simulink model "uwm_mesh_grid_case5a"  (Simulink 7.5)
settings: Solver=ode45  StartTime=0.0  StopTime=3.0  RelTol=1e-4
undefined symbols (not defined in the file or in its folder): D1, Delta, dfilt, DiscIntNeverNeededParam, Discrete, no, powergui, steady, ZData
libraries: powerlib x259, powerlib_extras x68, dsparch4 x11
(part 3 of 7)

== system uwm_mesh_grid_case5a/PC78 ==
  3-phase  Instantaneous  Active & Reactive Power : powerlib_extras/Measurements/3-phase  Instantaneous  Active & Reactive Power  DialogController=POWERSYS.PowerSysDialog  SystemSampleTime=-1
  Ground : powerlib/Elements/Ground  DialogController=POWERSYS.PowerSysDialog  PhysicalDomain=powersysdomain  SubClassName=unknown  LeftPortType=p1  RightPortType=p1  LConnTagsString=a
  Three-Phase Parallel RLC Branch : powerlib/Elements/Three-Phase Parallel RLC Branch  DialogController=POWERSYS.PowerSysDialog  PhysicalDomain=powersysdomain  SubClassName=unknown  LeftPortType=p1  RightPortType=p1  LConnTagsString=A|B|C  RConnTagsString=A|B|C  BranchType=C  Resistance=1  Inductance=1e-3  Capacitance=1/(C*2*pi*60)  Measurements=None
  Three-Phase Series RLC Branch3 : powerlib/Elements/Three-Phase Series RLC Branch  DialogController=POWERSYS.PowerSysDialog  PhysicalDomain=powersysdomain  SubClassName=unknown  LeftPortType=p1  RightPortType=p1  LConnTagsString=A|B|C  RConnTagsString=A|B|C  BranchType=RL  Resistance=R  Inductance=L/(2*pi*60)  Capacitance=1/(336*2*pi*60)  Measurements=None
  Three-Phase V-I Measurement : powerlib/Measurements/Three-Phase V-I Measurement  DialogController=POWERSYS.PowerSysDialog  SystemSampleTime=-1  VoltageMeasurement=phase-to-ground  SetLabelV=off  LabelV=Vabc  Vpu=off  VpuLL=off  CurrentMeasurement=yes  SetLabelI=off  LabelI=Iabc  Ipu=off  Pbase=100e6  Vbase=500e3  OutputType=Complex  PhasorSimulation=off  PSBequivalent=0
  A* : PMIOPort  Tag=PMCPort  Port=1  Side=Right
  B* : PMIOPort  Tag=PMCPort  Port=2  Side=Right
  C* : PMIOPort  Tag=PMCPort  Port=3  Side=Right
  A : PMIOPort  Tag=PMCPort  Port=4  Side=Left
  B : PMIOPort  Tag=PMCPort  Port=5  Side=Left
  C : PMIOPort  Tag=PMCPort  Port=6  Side=Left
  PQ : Outport  OutDataType=fixdt(1, 16)  OutScaling=2^0
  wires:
  Three-Phase V-I Measurement/1 -> 3-phase  Instantaneous  Active & Reactive Power/1
  Three-Phase V-I Measurement/2 -> 3-phase  Instantaneous  Active & Reactive Power/2
  3-phase  Instantaneous  Active & Reactive Power/1 -> PQ/1
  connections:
  Three-Phase Parallel RLC Branch/LConn1 -- A*/RConn1 -- Three-Phase Series RLC Branch3/LConn1
  Three-Phase Parallel RLC Branch/LConn2 -- B*/RConn1 -- Three-Phase Series RLC Branch3/LConn2
  Three-Phase Parallel RLC Branch/LConn3 -- C*/RConn1 -- Three-Phase Series RLC Branch3/LConn3
  Ground/LConn1 -- Three-Phase Parallel RLC Branch/RConn2 -- Three-Phase Parallel RLC Branch/RConn1 -- Three-Phase Parallel RLC Branch/RConn3
  Three-Phase V-I Measurement/RConn2 -- Three-Phase Series RLC Branch3/RConn2
  Three-Phase V-I Measurement/RConn3 -- Three-Phase Series RLC Branch3/RConn3
  Three-Phase V-I Measurement/RConn1 -- Three-Phase Series RLC Branch3/RConn1
  A/RConn1 -- Three-Phase V-I Measurement/LConn1
  B/RConn1 -- Three-Phase V-I Measurement/LConn2
  C/RConn1 -- Three-Phase V-I Measurement/LConn3

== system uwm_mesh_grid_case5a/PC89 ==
  3-phase  Instantaneous  Active & Reactive Power : powerlib_extras/Measurements/3-phase  Instantaneous  Active & Reactive Power  DialogController=POWERSYS.PowerSysDialog  SystemSampleTime=-1
  Ground : powerlib/Elements/Ground  DialogController=POWERSYS.PowerSysDialog  PhysicalDomain=powersysdomain  SubClassName=unknown  LeftPortType=p1  RightPortType=p1  LConnTagsString=a
  Three-Phase Parallel RLC Branch : powerlib/Elements/Three-Phase Parallel RLC Branch  DialogController=POWERSYS.PowerSysDialog  PhysicalDomain=powersysdomain  SubClassName=unknown  LeftPortType=p1  RightPortType=p1  LConnTagsString=A|B|C  RConnTagsString=A|B|C  BranchType=C  Resistance=1  Inductance=1e-3  Capacitance=1/(C*2*pi*60)  Measurements=None
  Three-Phase Series RLC Branch3 : powerlib/Elements/Three-Phase Series RLC Branch  DialogController=POWERSYS.PowerSysDialog  PhysicalDomain=powersysdomain  SubClassName=unknown  LeftPortType=p1  RightPortType=p1  LConnTagsString=A|B|C  RConnTagsString=A|B|C  BranchType=RL  Resistance=R  Inductance=L/(2*pi*60)  Capacitance=1/(336*2*pi*60)  Measurements=None
  Three-Phase V-I Measurement : powerlib/Measurements/Three-Phase V-I Measurement  DialogController=POWERSYS.PowerSysDialog  SystemSampleTime=-1  VoltageMeasurement=phase-to-ground  SetLabelV=off  LabelV=Vabc  Vpu=off  VpuLL=off  CurrentMeasurement=yes  SetLabelI=off  LabelI=Iabc  Ipu=off  Pbase=100e6  Vbase=500e3  OutputType=Complex  PhasorSimulation=off  PSBequivalent=0
  A* : PMIOPort  Tag=PMCPort  Port=1  Side=Right
  B* : PMIOPort  Tag=PMCPort  Port=2  Side=Right
  C* : PMIOPort  Tag=PMCPort  Port=3  Side=Right
  A : PMIOPort  Tag=PMCPort  Port=4  Side=Left
  B : PMIOPort  Tag=PMCPort  Port=5  Side=Left
  C : PMIOPort  Tag=PMCPort  Port=6  Side=Left
  PQ : Outport  OutDataType=fixdt(1, 16)  OutScaling=2^0
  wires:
  Three-Phase V-I Measurement/1 -> 3-phase  Instantaneous  Active & Reactive Power/1
  Three-Phase V-I Measurement/2 -> 3-phase  Instantaneous  Active & Reactive Power/2
  3-phase  Instantaneous  Active & Reactive Power/1 -> PQ/1
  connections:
  Three-Phase Parallel RLC Branch/LConn1 -- A*/RConn1 -- Three-Phase Series RLC Branch3/LConn1
  Three-Phase Parallel RLC Branch/LConn2 -- B*/RConn1 -- Three-Phase Series RLC Branch3/LConn2
  Three-Phase Parallel RLC Branch/LConn3 -- C*/RConn1 -- Three-Phase Series RLC Branch3/LConn3
  Ground/LConn1 -- Three-Phase Parallel RLC Branch/RConn2 -- Three-Phase Parallel RLC Branch/RConn1 -- Three-Phase Parallel RLC Branch/RConn3
  Three-Phase V-I Measurement/RConn2 -- Three-Phase Series RLC Branch3/RConn2
  Three-Phase V-I Measurement/RConn3 -- Three-Phase Series RLC Branch3/RConn3
  Three-Phase V-I Measurement/RConn1 -- Three-Phase Series RLC Branch3/RConn1
  A/RConn1 -- Three-Phase V-I Measurement/LConn1
  B/RConn1 -- Three-Phase V-I Measurement/LConn2
  C/RConn1 -- Three-Phase V-I Measurement/LConn3

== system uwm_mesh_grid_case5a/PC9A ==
  3-phase  Instantaneous  Active & Reactive Power : powerlib_extras/Measurements/3-phase  Instantaneous  Active & Reactive Power  DialogController=POWERSYS.PowerSysDialog  SystemSampleTime=-1
  Ground : powerlib/Elements/Ground  DialogController=POWERSYS.PowerSysDialog  PhysicalDomain=powersysdomain  SubClassName=unknown  LeftPortType=p1  RightPortType=p1  LConnTagsString=a
  Three-Phase Parallel RLC Branch : powerlib/Elements/Three-Phase Parallel RLC Branch  DialogController=POWERSYS.PowerSysDialog  PhysicalDomain=powersysdomain  SubClassName=unknown  LeftPortType=p1  RightPortType=p1  LConnTagsString=A|B|C  RConnTagsString=A|B|C  BranchType=C  Resistance=1  Inductance=1e-3  Capacitance=1/(C*2*pi*60)  Measurements=None
  Three-Phase Series RLC Branch3 : powerlib/Elements/Three-Phase Series RLC Branch  DialogController=POWERSYS.PowerSysDialog  PhysicalDomain=powersysdomain  SubClassName=unknown  LeftPortType=p1  RightPortType=p1  LConnTagsString=A|B|C  RConnTagsString=A|B|C  BranchType=RL  Resistance=R  Inductance=L/(2*pi*60)  Capacitance=1/(336*2*pi*60)  Measurements=None
  Three-Phase V-I Measurement : powerlib/Measurements/Three-Phase V-I Measurement  DialogController=POWERSYS.PowerSysDialog  SystemSampleTime=-1  VoltageMeasurement=phase-to-ground  SetLabelV=off  LabelV=Vabc  Vpu=off  VpuLL=off  CurrentMeasurement=yes  SetLabelI=off  LabelI=Iabc  Ipu=off  Pbase=100e6  Vbase=500e3  OutputType=Complex  PhasorSimulation=off  PSBequivalent=0
  A* : PMIOPort  Tag=PMCPort  Port=1  Side=Right
  B* : PMIOPort  Tag=PMCPort  Port=2  Side=Right
  C* : PMIOPort  Tag=PMCPort  Port=3  Side=Right
  A : PMIOPort  Tag=PMCPort  Port=4  Side=Left
  B : PMIOPort  Tag=PMCPort  Port=5  Side=Left
  C : PMIOPort  Tag=PMCPort  Port=6  Side=Left
  PQ : Outport  OutDataType=fixdt(1, 16)  OutScaling=2^0
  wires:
  Three-Phase V-I Measurement/1 -> 3-phase  Instantaneous  Active & Reactive Power/1
  Three-Phase V-I Measurement/2 -> 3-phase  Instantaneous  Active & Reactive Power/2
  3-phase  Instantaneous  Active & Reactive Power/1 -> PQ/1
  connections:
  Three-Phase Parallel RLC Branch/LConn1 -- A*/RConn1 -- Three-Phase Series RLC Branch3/LConn1
  Three-Phase Parallel RLC Branch/LConn2 -- B*/RConn1 -- Three-Phase Series RLC Branch3/LConn2
  Three-Phase Parallel RLC Branch/LConn3 -- C*/RConn1 -- Three-Phase Series RLC Branch3/LConn3
  Ground/LConn1 -- Three-Phase Parallel RLC Branch/RConn2 -- Three-Phase Parallel RLC Branch/RConn1 -- Three-Phase Parallel RLC Branch/RConn3
  Three-Phase V-I Measurement/RConn2 -- Three-Phase Series RLC Branch3/RConn2
  Three-Phase V-I Measurement/RConn3 -- Three-Phase Series RLC Branch3/RConn3
  Three-Phase V-I Measurement/RConn1 -- Three-Phase Series RLC Branch3/RConn1
  A/RConn1 -- Three-Phase V-I Measurement/LConn1
  B/RConn1 -- Three-Phase V-I Measurement/LConn2
  C/RConn1 -- Three-Phase V-I Measurement/LConn3

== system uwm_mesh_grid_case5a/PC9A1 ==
  3-phase  Instantaneous  Active & Reactive Power : powerlib_extras/Measurements/3-phase  Instantaneous  Active & Reactive Power  DialogController=POWERSYS.PowerSysDialog  SystemSampleTime=-1
  Ground : powerlib/Elements/Ground  DialogController=POWERSYS.PowerSysDialog  PhysicalDomain=powersysdomain  SubClassName=unknown  LeftPortType=p1  RightPortType=p1  LConnTagsString=a
  Three-Phase Parallel RLC Branch : powerlib/Elements/Three-Phase Parallel RLC Branch  DialogController=POWERSYS.PowerSysDialog  PhysicalDomain=powersysdomain  SubClassName=unknown  LeftPortType=p1  RightPortType=p1  LConnTagsString=A|B|C  RConnTagsString=A|B|C  BranchType=C  Resistance=1  Inductance=1e-3  Capacitance=1/(C*2*pi*60)  Measurements=None
  Three-Phase Series RLC Branch3 : powerlib/Elements/Three-Phase Series RLC Branch  DialogController=POWERSYS.PowerSysDialog  PhysicalDomain=powersysdomain  SubClassName=unknown  LeftPortType=p1  RightPortType=p1  LConnTagsString=A|B|C  RConnTagsString=A|B|C  BranchType=RL  Resistance=R  Inductance=L/(2*pi*60)  Capacitance=1/(336*2*pi*60)  Measurements=None
  Three-Phase V-I Measurement : powerlib/Measurements/Three-Phase V-I Measurement  DialogController=POWERSYS.PowerSysDialog  SystemSampleTime=-1  VoltageMeasurement=phase-to-ground  SetLabelV=off  LabelV=Vabc  Vpu=off  VpuLL=off  CurrentMeasurement=yes  SetLabelI=off  LabelI=Iabc  Ipu=off  Pbase=100e6  Vbase=500e3  OutputType=Complex  PhasorSimulation=off  PSBequivalent=0
  A* : PMIOPort  Tag=PMCPort  Port=1  Side=Right
  B* : PMIOPort  Tag=PMCPort  Port=2  Side=Right
  C* : PMIOPort  Tag=PMCPort  Port=3  Side=Right
  A : PMIOPort  Tag=PMCPort  Port=4  Side=Left
  B : PMIOPort  Tag=PMCPort  Port=5  Side=Left
  C : PMIOPort  Tag=PMCPort  Port=6  Side=Left
  PQ : Outport  OutDataType=fixdt(1, 16)  OutScaling=2^0
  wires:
  Three-Phase V-I Measurement/1 -> 3-phase  Instantaneous  Active & Reactive Power/1
  Three-Phase V-I Measurement/2 -> 3-phase  Instantaneous  Active & Reactive Power/2
  3-phase  Instantaneous  Active & Reactive Power/1 -> PQ/1
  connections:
  Three-Phase Parallel RLC Branch/LConn1 -- A*/RConn1 -- Three-Phase Series RLC Branch3/LConn1
  Three-Phase Parallel RLC Branch/LConn2 -- B*/RConn1 -- Three-Phase Series RLC Branch3/LConn2
  Three-Phase Parallel RLC Branch/LConn3 -- C*/RConn1 -- Three-Phase Series RLC Branch3/LConn3
  Ground/LConn1 -- Three-Phase Parallel RLC Branch/RConn2 -- Three-Phase Parallel RLC Branch/RConn1 -- Three-Phase Parallel RLC Branch/RConn3
  Three-Phase V-I Measurement/RConn2 -- Three-Phase Series RLC Branch3/RConn2
  Three-Phase V-I Measurement/RConn3 -- Three-Phase Series RLC Branch3/RConn3
  Three-Phase V-I Measurement/RConn1 -- Three-Phase Series RLC Branch3/RConn1
  A/RConn1 -- Three-Phase V-I Measurement/LConn1
  B/RConn1 -- Three-Phase V-I Measurement/LConn2
  C/RConn1 -- Three-Phase V-I Measurement/LConn3

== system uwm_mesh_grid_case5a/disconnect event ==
  Step1 : Step  Time=[tstart]  Before=1  After=0  SampleTime=0
  Step2 : Step  Time=[tstop]  SampleTime=0
  Sum : Sum  OutDataType=fixdt(1, 16)  OutScaling=2^0
  Out1 : Outport
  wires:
  Step2/1 -> Sum/2
  Step1/1 -> Sum/1
  Sum/1 -> Out1/1

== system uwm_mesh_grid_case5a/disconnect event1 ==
  Step1 : Step  Time=[tstart]  Before=1  After=0  SampleTime=0
  Step2 : Step  Time=[tstop]  SampleTime=0
  Sum : Sum  OutDataType=fixdt(1, 16)  OutScaling=2^0
  Out1 : Outport
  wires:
  Step2/1 -> Sum/2
  Step1/1 -> Sum/1
  Sum/1 -> Out1/1

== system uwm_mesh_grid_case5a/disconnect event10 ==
  Step1 : Step  Time=[tstart]  Before=1  After=0  SampleTime=0
  Step2 : Step  Time=[tstop]  SampleTime=0
  Sum : Sum  OutDataType=fixdt(1, 16)  OutScaling=2^0
  Out1 : Outport
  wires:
  Step2/1 -> Sum/2
  Step1/1 -> Sum/1
  Sum/1 -> Out1/1

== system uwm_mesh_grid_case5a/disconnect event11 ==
  Step1 : Step  Time=[tstart]  Before=1  After=0  SampleTime=0
  Step2 : Step  Time=[tstop]  SampleTime=0
  Sum : Sum  OutDataType=fixdt(1, 16)  OutScaling=2^0
  Out1 : Outport
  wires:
  Step2/1 -> Sum/2
  Step1/1 -> Sum/1
  Sum/1 -> Out1/1

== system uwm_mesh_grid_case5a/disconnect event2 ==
  Step1 : Step  Time=[tstart]  Before=1  After=0  SampleTime=0
  Step2 : Step  Time=[tstop]  SampleTime=0
  Sum : Sum  OutDataType=fixdt(1, 16)  OutScaling=2^0
  Out1 : Outport
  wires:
  Step2/1 -> Sum/2
  Step1/1 -> Sum/1
  Sum/1 -> Out1/1

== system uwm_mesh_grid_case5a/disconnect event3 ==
  Step1 : Step  Time=[tstart]  Before=1  After=0  SampleTime=0
  Step2 : Step  Time=[tstop]  SampleTime=0
  Sum : Sum  OutDataType=fixdt(1, 16)  OutScaling=2^0
  Out1 : Outport
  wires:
  Step2/1 -> Sum/2
  Step1/1 -> Sum/1
  Sum/1 -> Out1/1

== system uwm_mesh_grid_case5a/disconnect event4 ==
  Step1 : Step  Time=[tstart]  Before=1  After=0  SampleTime=0
  Step2 : Step  Time=[tstop]  SampleTime=0
  Sum : Sum  OutDataType=fixdt(1, 16)  OutScaling=2^0
  Out1 : Outport
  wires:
  Step2/1 -> Sum/2
  Step1/1 -> Sum/1
  Sum/1 -> Out1/1

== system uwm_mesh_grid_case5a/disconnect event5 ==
  Step1 : Step  Time=[tstart]  Before=1  After=0  SampleTime=0
  Step2 : Step  Time=[tstop]  SampleTime=0
  Sum : Sum  OutDataType=fixdt(1, 16)  OutScaling=2^0
  Out1 : Outport
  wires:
  Step2/1 -> Sum/2
  Step1/1 -> Sum/1
  Sum/1 -> Out1/1

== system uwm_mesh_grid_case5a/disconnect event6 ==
  Step1 : Step  Time=[tstart]  Before=1  After=0  SampleTime=0
  Step2 : Step  Time=[tstop]  SampleTime=0
  Sum : Sum  OutDataType=fixdt(1, 16)  OutScaling=2^0
  Out1 : Outport
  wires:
  Step2/1 -> Sum/2
  Step1/1 -> Sum/1
  Sum/1 -> Out1/1

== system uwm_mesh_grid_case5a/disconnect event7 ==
  Step1 : Step  Time=[tstart]  Before=1  After=0  SampleTime=0
  Step2 : Step  Time=[tstop]  SampleTime=0
  Sum : Sum  OutDataType=fixdt(1, 16)  OutScaling=2^0
  Out1 : Outport
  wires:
  Step2/1 -> Sum/2
  Step1/1 -> Sum/1
  Sum/1 -> Out1/1

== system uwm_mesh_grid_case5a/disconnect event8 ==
  Step1 : Step  Time=[tstart]  Before=1  After=0  SampleTime=0
  Step2 : Step  Time=[tstop]  SampleTime=0
  Sum : Sum  OutDataType=fixdt(1, 16)  OutScaling=2^0
  Out1 : Outport
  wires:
  Step2/1 -> Sum/2
  Step1/1 -> Sum/1
  Sum/1 -> Out1/1

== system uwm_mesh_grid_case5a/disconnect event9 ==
  Step1 : Step  Time=[tstart]  Before=1  After=0  SampleTime=0
  Step2 : Step  Time=[tstop]  SampleTime=0
  Sum : Sum  OutDataType=fixdt(1, 16)  OutScaling=2^0
  Out1 : Outport
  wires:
  Step2/1 -> Sum/2
  Step1/1 -> Sum/1
  Sum/1 -> Out1/1

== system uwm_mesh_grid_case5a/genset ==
  Ereq : Inport  OutDataType=fixdt(1, 16)  OutScaling=2^0
  Preq : Inport  Port=2  OutDataType=fixdt(1, 16)  OutScaling=2^0
  3-phase  Instantaneous  Active & Reactive Power : powerlib_extras/Measurements/3-phase  Instantaneous  Active & Reactive Power  DialogController=POWERSYS.PowerSysDialog  SystemSampleTime=-1
  Bus Selector : BusSelector  OutputSignals="Mechanical.Rotor speed  wm  (pu)"
  Gain : Gain  Gain=60  ParameterDataType=fixdt(1, 16)  ParameterScaling=2^0  OutDataType=fixdt(1, 16)  OutScaling=2^0
  Ground : powerlib/Elements/Ground  DialogController=POWERSYS.PowerSysDialog  PhysicalDomain=powersysdomain  SubClassName=unknown  LeftPortType=p1  RightPortType=p1  LConnTagsString=a
  Mux : Mux  Inputs=2
  RMS block : Fcn  Expr=sqrt(u(1)*u(1)+u(2)*u(2)+u(3)*u(3))/sqrt(3)
  RMS block2 : Fcn  Expr=sqrt(u(1)*u(1)+u(2)*u(2)+u(3)*u(3))/sqrt(3)
  Synchronous Machine pu Standard : powerlib/Machines/Synchronous Machine pu Standard  DialogController=POWERSYS.PowerSysDialog  SystemSampleTime=-1  PresetModel=No  MechanicalLoad=Mechanical power Pm  ShowDetailedParameters=on  RotorType=Salient-pole  NominalParameters="[ 12500  208   60]"  Reactances1=[ 1.81, 0.3, 0.23, 1.76, 0.65, 0.25, 0.15 ]  Reactances2="[ 1.204, 0.125, 0.056, 0.533,  0.051,  0.037 ]"  dAxisTimeConstants=Short-circuit  qAxisTimeConstants=Short-circuit  TimeConstants1="[ 4.4849  0.0681  0.1  ]"  TimeConstants2=[ 8.0, 0.03, 1.0, 0.07 ]  TimeConstants3="[  .35523  0.00015  0.067  ]"  TimeConstants4=[ 8.0, 0.03, 0.3371, 0.0295 ]  TimeConstants5=[ 1.01, 0.053, 0.1 ]  TimeConstants6=[ 1.3201, 0.023, 1.0, 0.07 ]  TimeConstants7=[0.35523 0.00015 0.0067]  TimeConstants8=[ 1.3201, 0.0231, 0.3371, 0.0295 ]  StatorResistance=0.0217  Mechanical=[ .19 0 2 ]  PolePairs=2  InitialConditions="[ 0  0  0  0  0  0  0  0  1 ]"  SetSaturation=off  Saturation=[0.6404,0.7127,0.8441,0.9214,0.9956,1.082,1.19,1.316,1.457;0.7,0.7698,0.8872,0.9466,0.9969,1.046,1.1,1.151,1.201]  Units=per unit standard parameters  LoadFlowParameters=[1 0 0 0 0]  TsPowergui=0  TsBlock=-1  IterativeModel=Forward Euler
  T1 : powerlib/Elements/Three-Phase Transformer (Two Windings)  DialogController=POWERSYS.PowerSysDialog  SystemSampleTime=-1  Winding1Connection=Delta (D1)  UNITS=SI  NominalPower=[ 45e3 , 60 ]  Winding1=[208 .02688 .10752/(2*pi*60)]  Winding2Connection=Yg  Winding2=[208 .005047 .201899/(2*pi*60)]  SetSaturation=off  Rm=1e+08  Lm=7650.8  Saturation=[0 0;1359.8 0.93633;5.6659e+05 1.186]  Hysteresis=off  DataFile='hysteresis'  SetInitialFlux=off  InitialFluxes=[0.62422 -0.62422 0.54618]  Measurements=None  MoreParameters=off  BreakLoop=off  DataType=on  TransfoNumber=1
  Three-Phase Series RLC Branch : powerlib/Elements/Three-Phase Series RLC Branch  DialogController=POWERSYS.PowerSysDialog  PhysicalDomain=powersysdomain  SubClassName=unknown  LeftPortType=p1  RightPortType=p1  LConnTagsString=A|B|C  RConnTagsString=A|B|C  BranchType=C  Resistance=1  Inductance=1e-3  Capacitance=1.e-4  Measurements=None
  Three-Phase V-I Measurement : powerlib/Measurements/Three-Phase V-I Measurement  DialogController=POWERSYS.PowerSysDialog  SystemSampleTime=-1  VoltageMeasurement=phase-to-ground  SetLabelV=off  LabelV=Vabc  Vpu=off  VpuLL=off  CurrentMeasurement=yes  SetLabelI=off  LabelI=Iabc  Ipu=off  Pbase=100e6  Vbase=500e3  OutputType=Complex  PhasorSimulation=off  PSBequivalent=0
  genset  controller : Subsystem  mask{Vbase=208, Sbase=12500}
  a : PMIOPort  Port=1  Side=Right
  b : PMIOPort  Port=2  Side=Right
  c : PMIOPort  Port=3  Side=Right
  PQ : Outport  OutDataType=fixdt(1, 16)  OutScaling=2^0
  V : Outport  Port=2  OutDataType=fixdt(1, 16)  OutScaling=2^0
  I : Outport  Port=3  OutDataType=fixdt(1, 16)  OutScaling=2^0
  RMS : Outport  Port=4  OutDataType=fixdt(1, 16)  OutScaling=2^0
  freq : Outport  Port=5  OutDataType=fixdt(1, 16)  OutScaling=2^0
  Pmm : Outport  Port=6
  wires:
  genset  controller/1(Pmech) -> Synchronous Machine pu Standard/1  "Pmec (pu)"
  genset  controller/2(Vf) -> Synchronous Machine pu Standard/2  "Vf (pu)"
  Synchronous Machine pu Standard/1 -> Bus Selector/1
  Bus Selector/1 -> genset  controller/1(wr)  "<Rotor speed  wm  (pu)>"
  Three-Phase V-I Measurement/1 -> genset  controller/2(Vabc), 3-phase  Instantaneous  Active & Reactive Power/1, RMS block2/1, V/1
  Three-Phase V-I Measurement/2 -> genset  controller/3(Iabc), 3-phase  Instantaneous  Active & Reactive Power/2, RMS block/1, I/1
  Preq/1 -> genset  controller/4(Preq)
  Ereq/1 -> genset  controller/5(Ereq1)
  genset  controller/3(w) -> Gain/1
  Gain/1 -> freq/1
  3-phase  Instantaneous  Active & Reactive Power/1 -> PQ/1
  RMS block2/1 -> Mux/1
  RMS block/1 -> Mux/2
  Mux/1 -> RMS/1
  genset  controller/4(Pmm) -> Pmm/1
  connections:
  Three-Phase Series RLC Branch/RConn2 -- Three-Phase Series RLC Branch/RConn1 -- Ground/LConn1 -- Three-Phase Series RLC Branch/RConn3
  Synchronous Machine pu Standard/RConn1 -- T1/LConn1 -- Three-Phase Series RLC Branch/LConn1
  Synchronous Machine pu Standard/RConn2 -- T1/LConn2 -- Three-Phase Series RLC Branch/LConn2
  Synchronous Machine pu Standard/RConn3 -- T1/LConn3 -- Three-Phase Series RLC Branch/LConn3
  T1/RConn2 -- Three-Phase V-I Measurement/LConn2
  T1/RConn1 -- Three-Phase V-I Measurement/LConn1
  T1/RConn3 -- Three-Phase V-I Measurement/LConn3
  Three-Phase V-I Measurement/RConn1 -- a/RConn1
  b/RConn1 -- Three-Phase V-I Measurement/RConn2
  c/RConn1 -- Three-Phase V-I Measurement/RConn3

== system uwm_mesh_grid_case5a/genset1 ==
  Ereq : Inport  OutDataType=fixdt(1, 16)  OutScaling=2^0
  Preq : Inport  Port=2  OutDataType=fixdt(1, 16)  OutScaling=2^0
  3-phase  Instantaneous  Active & Reactive Power : powerlib_extras/Measurements/3-phase  Instantaneous  Active & Reactive Power  DialogController=POWERSYS.PowerSysDialog  SystemSampleTime=-1
  Bus Selector : BusSelector  OutputSignals="Mechanical.Rotor speed  wm  (pu)"
  Gain : Gain  Gain=60  ParameterDataType=fixdt(1, 16)  ParameterScaling=2^0  OutDataType=fixdt(1, 16)  OutScaling=2^0
  Ground : powerlib/Elements/Ground  DialogController=POWERSYS.PowerSysDialog  PhysicalDomain=powersysdomain  SubClassName=unknown  LeftPortType=p1  RightPortType=p1  LConnTagsString=a
  Mux : Mux  Inputs=2
  RMS block : Fcn  Expr=sqrt(u(1)*u(1)+u(2)*u(2)+u(3)*u(3))/sqrt(3)
  RMS block2 : Fcn  Expr=sqrt(u(1)*u(1)+u(2)*u(2)+u(3)*u(3))/sqrt(3)
  Synchronous Machine pu Standard : powerlib/Machines/Synchronous Machine pu Standard  DialogController=POWERSYS.PowerSysDialog  SystemSampleTime=-1  PresetModel=No  MechanicalLoad=Mechanical power Pm  ShowDetailedParameters=on  RotorType=Salient-pole  NominalParameters="[ 12500  208   60]"  Reactances1=[ 1.81, 0.3, 0.23, 1.76, 0.65, 0.25, 0.15 ]  Reactances2="[ 1.204, 0.125, 0.056, 0.533,  0.051,  0.037 ]"  dAxisTimeConstants=Short-circuit  qAxisTimeConstants=Short-circuit  TimeConstants1="[ 4.4849  0.0681  0.1  ]"  TimeConstants2=[ 8.0, 0.03, 1.0, 0.07 ]  TimeConstants3="[  .35523  0.00015  0.067  ]"  TimeConstants4=[ 8.0, 0.03, 0.3371, 0.0295 ]  TimeConstants5=[ 1.01, 0.053, 0.1 ]  TimeConstants6=[ 1.3201, 0.023, 1.0, 0.07 ]  TimeConstants7=[0.35523 0.00015 0.0067]  TimeConstants8=[ 1.3201, 0.0231, 0.3371, 0.0295 ]  StatorResistance=0.0217  Mechanical=[ .19 0 2 ]  PolePairs=2  InitialConditions="[ 0  0  0  0  0  0  0  0  1 ]"  SetSaturation=off  Saturation=[0.6404,0.7127,0.8441,0.9214,0.9956,1.082,1.19,1.316,1.457;0.7,0.7698,0.8872,0.9466,0.9969,1.046,1.1,1.151,1.201]  Units=per unit standard parameters  LoadFlowParameters=[1 0 0 0 0]  TsPowergui=0  TsBlock=-1  IterativeModel=Forward Euler
  T1 : powerlib/Elements/Three-Phase Transformer (Two Windings)  DialogController=POWERSYS.PowerSysDialog  SystemSampleTime=-1  Winding1Connection=Delta (D1)  UNITS=SI  NominalPower=[ 45e3 , 60 ]  Winding1=[208 .02688 .10752/(2*pi*60)]  Winding2Connection=Yg  Winding2=[208 .005047 .201899/(2*pi*60)]  SetSaturation=off  Rm=1e+08  Lm=7650.8  Saturation=[0 0;1359.8 0.93633;5.6659e+05 1.186]  Hysteresis=off  DataFile='hysteresis'  SetInitialFlux=off  InitialFluxes=[0.62422 -0.62422 0.54618]  Measurements=None  MoreParameters=off  BreakLoop=off  DataType=on  TransfoNumber=1
  Three-Phase Series RLC Branch : powerlib/Elements/Three-Phase Series RLC Branch  DialogController=POWERSYS.PowerSysDialog  PhysicalDomain=powersysdomain  SubClassName=unknown  LeftPortType=p1  RightPortType=p1  LConnTagsString=A|B|C  RConnTagsString=A|B|C  BranchType=C  Resistance=1  Inductance=1e-3  Capacitance=1.e-4  Measurements=None
  Three-Phase V-I Measurement : powerlib/Measurements/Three-Phase V-I Measurement  DialogController=POWERSYS.PowerSysDialog  SystemSampleTime=-1  VoltageMeasurement=phase-to-ground  SetLabelV=off  LabelV=Vabc  Vpu=off  VpuLL=off  CurrentMeasurement=yes  SetLabelI=off  LabelI=Iabc  Ipu=off  Pbase=100e6  Vbase=500e3  OutputType=Complex  PhasorSimulation=off  PSBequivalent=0
  genset  controller : Subsystem  mask{Vbase=208, Sbase=12500}
  a : PMIOPort  Port=1  Side=Right
  b : PMIOPort  Port=2  Side=Right
  c : PMIOPort  Port=3  Side=Right
  PQ : Outport  OutDataType=fixdt(1, 16)  OutScaling=2^0
  V : Outport  Port=2  OutDataType=fixdt(1, 16)  OutScaling=2^0
  I : Outport  Port=3  OutDataType=fixdt(1, 16)  OutScaling=2^0
  RMS : Outport  Port=4  OutDataType=fixdt(1, 16)  OutScaling=2^0
  freq : Outport  Port=5  OutDataType=fixdt(1, 16)  OutScaling=2^0
  Pmm : Outport  Port=6
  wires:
  genset  controller/1(Pmech) -> Synchronous Machine pu Standard/1  "Pmec (pu)"
  genset  controller/2(Vf) -> Synchronous Machine pu Standard/2  "Vf (pu)"
  Synchronous Machine pu Standard/1 -> Bus Selector/1
  Bus Selector/1 -> genset  controller/1(wr)  "<Rotor speed  wm  (pu)>"
  Three-Phase V-I Measurement/1 -> genset  controller/2(Vabc), 3-phase  Instantaneous  Active & Reactive Power/1, RMS block2/1, V/1
  Three-Phase V-I Measurement/2 -> genset  controller/3(Iabc), 3-phase  Instantaneous  Active & Reactive Power/2, RMS block/1, I/1
  Preq/1 -> genset  controller/4(Preq)
  Ereq/1 -> genset  controller/5(Ereq1)
  genset  controller/3(w) -> Gain/1
  Gain/1 -> freq/1
  3-phase  Instantaneous  Active & Reactive Power/1 -> PQ/1
  RMS block2/1 -> Mux/1
  RMS block/1 -> Mux/2
  Mux/1 -> RMS/1
  genset  controller/4(Pmm) -> Pmm/1
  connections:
  Three-Phase Series RLC Branch/RConn2 -- Three-Phase Series RLC Branch/RConn1 -- Ground/LConn1 -- Three-Phase Series RLC Branch/RConn3
  Synchronous Machine pu Standard/RConn1 -- T1/LConn1 -- Three-Phase Series RLC Branch/LConn1
  Synchronous Machine pu Standard/RConn2 -- T1/LConn2 -- Three-Phase Series RLC Branch/LConn2
  Synchronous Machine pu Standard/RConn3 -- T1/LConn3 -- Three-Phase Series RLC Branch/LConn3
  T1/RConn2 -- Three-Phase V-I Measurement/LConn2
  T1/RConn1 -- Three-Phase V-I Measurement/LConn1
  T1/RConn3 -- Three-Phase V-I Measurement/LConn3
  Three-Phase V-I Measurement/RConn1 -- a/RConn1
  b/RConn1 -- Three-Phase V-I Measurement/RConn2
  c/RConn1 -- Three-Phase V-I Measurement/RConn3

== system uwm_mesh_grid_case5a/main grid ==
  4.16kV 2500kVA : powerlib/Electrical Sources/Three-Phase Source  DialogController=POWERSYS.PowerSysDialog  SystemSampleTime=-1  Voltage=4160  PhaseAngle=0  Frequency=60  InternalConnection=Yg  SpecifyImpedance=on  Resistance=25^2/1000/10  Inductance=25^2/1000/377  ShortCircuitLevel=1200e6  BaseVoltage=4160  XRratio=100
  PC1 : Subsystem  mask{R=.093400, L=.025500, C=2894.3}
  T1 : powerlib/Elements/Three-Phase Transformer (Two Windings)  DialogController=POWERSYS.PowerSysDialog  SystemSampleTime=-1  Winding1Connection=Delta (D1)  UNITS=SI  NominalPower=[ 2500e3 , 60 ]  Winding1=[4160 .04706 .1882/(2*pi*60)]  Winding2Connection=Yg  Winding2=[480 .000627 .0025068/(2*pi*60)]  SetSaturation=off  Rm=1.e6  Lm=1.e6  Saturation=[0 0;589.26 2.1608;2.4552e+05 2.737]  Hysteresis=off  DataFile='hysteresis'  SetInitialFlux=off  InitialFluxes=[1.4405 -1.4405 1.2604]  Measurements=None  MoreParameters=off  BreakLoop=off  DataType=on  TransfoNumber=1
  T2 : powerlib/Elements/Three-Phase Transformer (Two Windings)  DialogController=POWERSYS.PowerSysDialog  SystemSampleTime=-1  Winding1Connection=Delta (D1)  UNITS=SI  NominalPower=[ 75e3 , 60 ]  Winding1=[480 .0169 .0676/(2*pi*60)]  Winding2Connection=Yg  Winding2=[208 .0003 .0127/(2*pi*60)]  SetSaturation=off  Rm=1.e6  Lm=1.e6  Saturation=[0 0;589.26 2.1608;2.4552e+05 2.737]  Hysteresis=off  DataFile='hysteresis'  SetInitialFlux=off  InitialFluxes=[1.4405 -1.4405 1.2604]  Measurements=None  MoreParameters=off  BreakLoop=off  DataType=on  TransfoNumber=1
  A : PMIOPort  Port=1  Side=Right
  B : PMIOPort  Port=2  Side=Right
  C : PMIOPort  Port=3  Side=Right
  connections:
  A/RConn1 -- T2/RConn1
  B/RConn1 -- T2/RConn2
  C/RConn1 -- T2/RConn3
  T1/RConn1 -- PC1/LConn1
  T1/RConn2 -- PC1/LConn2
  T1/RConn3 -- PC1/LConn3
  PC1/RConn1 -- T2/LConn1
  PC1/RConn2 -- T2/LConn2
  PC1/RConn3 -- T2/LConn3
  4.16kV 2500kVA/RConn2 -- T1/LConn2
  4.16kV 2500kVA/RConn1 -- T1/LConn1
  4.16kV 2500kVA/RConn3 -- T1/LConn3

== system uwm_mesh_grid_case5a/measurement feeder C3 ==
  3-phase  Instantaneous  Active & Reactive Power : powerlib_extras/Measurements/3-phase  Instantaneous  Active & Reactive Power  DialogController=POWERSYS.PowerSysDialog  SystemSampleTime=-1
  Ground : powerlib/Elements/Ground  DialogController=POWERSYS.PowerSysDialog  PhysicalDomain=powersysdomain  SubClassName=unknown  LeftPortType=p1  RightPortType=p1  LConnTagsString=a
  Mux : Mux  Inputs=2
  RMS block : Fcn  Expr=sqrt(u(1)*u(1)+u(2)*u(2)+u(3)*u(3))/sqrt(3)
  RMS block1 : Fcn  Expr=sqrt(u(1)*u(1)+u(2)*u(2)+u(3)*u(3))/sqrt(3)
  Three-Phase V-I Measurement : powerlib/Measurements/Three-Phase V-I Measurement  DialogController=POWERSYS.PowerSysDialog  SystemSampleTime=-1  VoltageMeasurement=phase-to-ground  SetLabelV=off  LabelV=Vabc  Vpu=off  VpuLL=off  CurrentMeasurement=yes  SetLabelI=off  LabelI=Iabc  Ipu=off  Pbase=100e6  Vbase=500e3  OutputType=Complex  PhasorSimulation=off  PSBequivalent=0
  Voltage  Measurement : powerlib/Measurements/Voltage Measurement  DialogController=POWERSYS.PowerSysDialog  SystemSampleTime=-1  PhasorSimulation=off  OutputType=Complex  PSBequivalent=0
  frequency estimator (discrete) : Subsystem  mask{dt=0.010}
      mask prompts: dt "sample time"
  A : PMIOPort  Port=1  Side=Left
  B : PMIOPort  Port=2  Side=Left
  a : PMIOPort  Port=3  Side=Right
  b : PMIOPort  Port=4  Side=Right
  C : PMIOPort  Port=5  Side=Left
  c : PMIOPort  Port=6  Side=Right
  PQ : Outport  OutDataType=fixdt(1, 16)  OutScaling=2^0
  V : Outport  Port=2  OutDataType=fixdt(1, 16)  OutScaling=2^0
  I : Outport  Port=3  OutDataType=fixdt(1, 16)  OutScaling=2^0
  RMS : Outport  Port=4  OutDataType=fixdt(1, 16)  OutScaling=2^0
  freq : Outport  Port=5  OutDataType=fixdt(1, 16)  OutScaling=2^0
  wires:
  Three-Phase V-I Measurement/1 -> 3-phase  Instantaneous  Active & Reactive Power/1, RMS block1/1, V/1
  Three-Phase V-I Measurement/2 -> 3-phase  Instantaneous  Active & Reactive Power/2, RMS block/1, I/1
  3-phase  Instantaneous  Active & Reactive Power/1 -> PQ/1
  RMS block1/1 -> Mux/1
  RMS block/1 -> Mux/2
  Mux/1 -> RMS/1
  Voltage  Measurement/1 -> frequency estimator (discrete)/1(v)
  frequency estimator (discrete)/1(w) -> freq/1
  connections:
  c/RConn1 -- Three-Phase V-I Measurement/RConn3
  C/RConn1 -- Three-Phase V-I Measurement/LConn3
  b/RConn1 -- Three-Phase V-I Measurement/RConn2
  a/RConn1 -- Three-Phase V-I Measurement/RConn1 -- Voltage  Measurement/LConn1
  B/RConn1 -- Three-Phase V-I Measurement/LConn2
  A/RConn1 -- Three-Phase V-I Measurement/LConn1
  Voltage  Measurement/LConn2 -- Ground/LConn1

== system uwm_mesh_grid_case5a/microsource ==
  E_req : Inport
  P_req : Inport  Port=2
  10 mH : powerlib/Elements/Three-Phase Series RLC Branch  DialogController=POWERSYS.PowerSysDialog  PhysicalDomain=powersysdomain  SubClassName=unknown  LeftPortType=p1  RightPortType=p1  LConnTagsString=A|B|C  RConnTagsString=A|B|C  BranchType=L  Resistance=.0028  Inductance=5e-3  Capacitance=1e-6  Measurements=None
  3-phase  Instantaneous  Active & Reactive Power : powerlib_extras/Measurements/3-phase  Instantaneous  Active & Reactive Power  DialogController=POWERSYS.PowerSysDialog  SystemSampleTime=-1
  Gain : Gain  Gain=1/(2*pi)  ParameterDataType=fixdt(1, 16)  ParameterScaling=2^0  OutDataType=fixdt(1, 16)  OutScaling=2^0
  Mux : Mux  Inputs=2
  RMS block : Fcn  Expr=sqrt(u(1)*u(1)+u(2)*u(2)+u(3)*u(3))/sqrt(3)
  RMS block1 : Fcn  Expr=sqrt(u(1)*u(1)+u(2)*u(2)+u(3)*u(3))/sqrt(3)
  T1 : powerlib/Elements/Three-Phase Transformer (Two Windings)  DialogController=POWERSYS.PowerSysDialog  SystemSampleTime=-1  Winding1Connection=Delta (D1)  UNITS=SI  NominalPower=[ 45e3 , 60 ]  Winding1=[208 0.02688 0.1075/(2*pi*60)]  Winding2Connection=Yg  Winding2=[208 0.005047 .0201/(2*pi*60)]  SetSaturation=off  Rm=100.e6  Lm=7650.8  Saturation=[0 0;1359.8 0.93633;5.6659e+05 1.186]  Hysteresis=off  DataFile='hysteresis'  SetInitialFlux=off  InitialFluxes=[0.62422 -0.62422 0.54618]  Measurements=None  MoreParameters=off  BreakLoop=off  DataType=on  TransfoNumber=1
  Three-Phase V-I Measurement : powerlib/Measurements/Three-Phase V-I Measurement  DialogController=POWERSYS.PowerSysDialog  SystemSampleTime=-1  VoltageMeasurement=phase-to-ground  SetLabelV=off  LabelV=Vabc  Vpu=off  VpuLL=off  CurrentMeasurement=yes  SetLabelI=off  LabelI=Iabc  Ipu=off  Pbase=100e6  Vbase=500e3  OutputType=Complex  PhasorSimulation=off  PSBequivalent=0
  UWM_controller : Subsystem  mask{Vbase=208, Sbase=15000}
  microsource : Subsystem
  a : PMIOPort  Port=1  Side=Right
  b : PMIOPort  Port=2  Side=Right
  c : PMIOPort  Port=3  Side=Right
  PQ : Outport  OutDataType=fixdt(1, 16)  OutScaling=2^0
  V : Outport  Port=2  OutDataType=fixdt(1, 16)  OutScaling=2^0
  I : Outport  Port=3  OutDataType=fixdt(1, 16)  OutScaling=2^0
  RMS : Outport  Port=4  OutDataType=fixdt(1, 16)  OutScaling=2^0
  freq : Outport  Port=5  OutDataType=fixdt(1, 16)  OutScaling=2^0
  Pmm : Outport  Port=6
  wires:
  E_req/1 -> UWM_controller/3(E_req)
  P_req/1 -> UWM_controller/4(P_req)
  Three-Phase V-I Measurement/1 -> UWM_controller/1(v_meas), 3-phase  Instantaneous  Active & Reactive Power/1, RMS block1/1, V/1
  Three-Phase V-I Measurement/2 -> UWM_controller/2(i_meas), 3-phase  Instantaneous  Active & Reactive Power/2, RMS block/1, I/1
  UWM_controller/1(Vpk) -> microsource/1(Vpk)
  UWM_controller/2(w) -> microsource/2(w), Gain/1
  Gain/1 -> freq/1
  3-phase  Instantaneous  Active & Reactive Power/1 -> PQ/1
  RMS block1/1 -> Mux/1
  RMS block/1 -> Mux/2
  Mux/1 -> RMS/1
  UWM_controller/3(Pmm) -> Pmm/1
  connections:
  b/RConn1 -- Three-Phase V-I Measurement/RConn2
  Three-Phase V-I Measurement/RConn3 -- c/RConn1
  10 mH/LConn2 -- microsource/RConn2
  10 mH/LConn1 -- microsource/RConn1
  10 mH/LConn3 -- microsource/RConn3
  T1/LConn1 -- 10 mH/RConn1
  T1/LConn2 -- 10 mH/RConn2
  T1/LConn3 -- 10 mH/RConn3
  T1/RConn1 -- Three-Phase V-I Measurement/LConn1
  T1/RConn2 -- Three-Phase V-I Measurement/LConn2
  T1/RConn3 -- Three-Phase V-I Measurement/LConn3
  a/RConn1 -- Three-Phase V-I Measurement/RConn1

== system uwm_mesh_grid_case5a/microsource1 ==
  E_req : Inport
  P_req : Inport  Port=2
  10 mH : powerlib/Elements/Three-Phase Series RLC Branch  DialogController=POWERSYS.PowerSysDialog  PhysicalDomain=powersysdomain  SubClassName=unknown  LeftPortType=p1  RightPortType=p1  LConnTagsString=A|B|C  RConnTagsString=A|B|C  BranchType=L  Resistance=.0028  Inductance=5e-3  Capacitance=1e-6  Measurements=None
  3-phase  Instantaneous  Active & Reactive Power : powerlib_extras/Measurements/3-phase  Instantaneous  Active & Reactive Power  DialogController=POWERSYS.PowerSysDialog  SystemSampleTime=-1
  Gain : Gain  Gain=1/(2*pi)  ParameterDataType=fixdt(1, 16)  ParameterScaling=2^0  OutDataType=fixdt(1, 16)  OutScaling=2^0
  Mux : Mux  Inputs=2
  RMS block : Fcn  Expr=sqrt(u(1)*u(1)+u(2)*u(2)+u(3)*u(3))/sqrt(3)
  RMS block1 : Fcn  Expr=sqrt(u(1)*u(1)+u(2)*u(2)+u(3)*u(3))/sqrt(3)
  T1 : powerlib/Elements/Three-Phase Transformer (Two Windings)  DialogController=POWERSYS.PowerSysDialog  SystemSampleTime=-1  Winding1Connection=Delta (D1)  UNITS=SI  NominalPower=[ 45e3 , 60 ]  Winding1=[208 0.02688 0.1075/(2*pi*60)]  Winding2Connection=Yg  Winding2=[208 0.005047 .0201/(2*pi*60)]  SetSaturation=off  Rm=100.e6  Lm=7650.8  Saturation=[0 0;1359.8 0.93633;5.6659e+05 1.186]  Hysteresis=off  DataFile='hysteresis'  SetInitialFlux=off  InitialFluxes=[0.62422 -0.62422 0.54618]  Measurements=None  MoreParameters=off  BreakLoop=off  DataType=on  TransfoNumber=1
  Three-Phase V-I Measurement : powerlib/Measurements/Three-Phase V-I Measurement  DialogController=POWERSYS.PowerSysDialog  SystemSampleTime=-1  VoltageMeasurement=phase-to-ground  SetLabelV=off  LabelV=Vabc  Vpu=off  VpuLL=off  CurrentMeasurement=yes  SetLabelI=off  LabelI=Iabc  Ipu=off  Pbase=100e6  Vbase=500e3  OutputType=Complex  PhasorSimulation=off  PSBequivalent=0
  UWM_controller : Subsystem  mask{Vbase=208, Sbase=15000}
  microsource : Subsystem
  a : PMIOPort  Port=1  Side=Right
  b : PMIOPort  Port=2  Side=Right
  c : PMIOPort  Port=3  Side=Right
  PQ : Outport  OutDataType=fixdt(1, 16)  OutScaling=2^0
  V : Outport  Port=2  OutDataType=fixdt(1, 16)  OutScaling=2^0
  I : Outport  Port=3  OutDataType=fixdt(1, 16)  OutScaling=2^0
  RMS : Outport  Port=4  OutDataType=fixdt(1, 16)  OutScaling=2^0
  freq : Outport  Port=5  OutDataType=fixdt(1, 16)  OutScaling=2^0
  Pmm : Outport  Port=6
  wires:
  E_req/1 -> UWM_controller/3(E_req)
  P_req/1 -> UWM_controller/4(P_req)
  Three-Phase V-I Measurement/1 -> UWM_controller/1(v_meas), 3-phase  Instantaneous  Active & Reactive Power/1, RMS block1/1, V/1
  Three-Phase V-I Measurement/2 -> UWM_controller/2(i_meas), 3-phase  Instantaneous  Active & Reactive Power/2, RMS block/1, I/1
  UWM_controller/1(Vpk) -> microsource/1(Vpk)
  UWM_controller/2(w) -> microsource/2(w), Gain/1
  Gain/1 -> freq/1
  3-phase  Instantaneous  Active & Reactive Power/1 -> PQ/1
  RMS block1/1 -> Mux/1
  RMS block/1 -> Mux/2
  Mux/1 -> RMS/1
  UWM_controller/3(Pmm) -> Pmm/1
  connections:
  b/RConn1 -- Three-Phase V-I Measurement/RConn2
  Three-Phase V-I Measurement/RConn3 -- c/RConn1
  10 mH/LConn2 -- microsource/RConn2
  10 mH/LConn1 -- microsource/RConn1
  10 mH/LConn3 -- microsource/RConn3
  T1/LConn1 -- 10 mH/RConn1
  T1/LConn2 -- 10 mH/RConn2
  T1/LConn3 -- 10 mH/RConn3
  T1/RConn1 -- Three-Phase V-I Measurement/LConn1
  T1/RConn2 -- Three-Phase V-I Measurement/LConn2
  T1/RConn3 -- Three-Phase V-I Measurement/LConn3
  a/RConn1 -- Three-Phase V-I Measurement/RConn1

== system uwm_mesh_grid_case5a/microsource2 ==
  E_req : Inport
  P_req : Inport  Port=2
  10 mH : powerlib/Elements/Three-Phase Series RLC Branch  DialogController=POWERSYS.PowerSysDialog  PhysicalDomain=powersysdomain  SubClassName=unknown  LeftPortType=p1  RightPortType=p1  LConnTagsString=A|B|C  RConnTagsString=A|B|C  BranchType=L  Resistance=.0028  Inductance=5e-3  Capacitance=1e-6  Measurements=None
  3-phase  Instantaneous  Active & Reactive Power : powerlib_extras/Measurements/3-phase  Instantaneous  Active & Reactive Power  DialogController=POWERSYS.PowerSysDialog  SystemSampleTime=-1
  Gain : Gain  Gain=1/(2*pi)  ParameterDataType=fixdt(1, 16)  ParameterScaling=2^0  OutDataType=fixdt(1, 16)  OutScaling=2^0
  Mux : Mux  Inputs=2
  RMS block : Fcn  Expr=sqrt(u(1)*u(1)+u(2)*u(2)+u(3)*u(3))/sqrt(3)
  RMS block1 : Fcn  Expr=sqrt(u(1)*u(1)+u(2)*u(2)+u(3)*u(3))/sqrt(3)
  T1 : powerlib/Elements/Three-Phase Transformer (Two Windings)  DialogController=POWERSYS.PowerSysDialog  SystemSampleTime=-1  Winding1Connection=Delta (D1)  UNITS=SI  NominalPower=[ 45e3 , 60 ]  Winding1=[208 0.02688 0.1075/(2*pi*60)]  Winding2Connection=Yg  Winding2=[208 0.005047 .0201/(2*pi*60)]  SetSaturation=off  Rm=100.e6  Lm=7650.8  Saturation=[0 0;1359.8 0.93633;5.6659e+05 1.186]  Hysteresis=off  DataFile='hysteresis'  SetInitialFlux=off  InitialFluxes=[0.62422 -0.62422 0.54618]  Measurements=None  MoreParameters=off  BreakLoop=off  DataType=on  TransfoNumber=1
  Three-Phase V-I Measurement : powerlib/Measurements/Three-Phase V-I Measurement  DialogController=POWERSYS.PowerSysDialog  SystemSampleTime=-1  VoltageMeasurement=phase-to-ground  SetLabelV=off  LabelV=Vabc  Vpu=off  VpuLL=off  CurrentMeasurement=yes  SetLabelI=off  LabelI=Iabc  Ipu=off  Pbase=100e6  Vbase=500e3  OutputType=Complex  PhasorSimulation=off  PSBequivalent=0
  UWM_controller : Subsystem  mask{Vbase=208, Sbase=15000}
  microsource : Subsystem
  a : PMIOPort  Port=1  Side=Right
  b : PMIOPort  Port=2  Side=Right
  c : PMIOPort  Port=3  Side=Right
  PQ : Outport  OutDataType=fixdt(1, 16)  OutScaling=2^0
  V : Outport  Port=2  OutDataType=fixdt(1, 16)  OutScaling=2^0
  I : Outport  Port=3  OutDataType=fixdt(1, 16)  OutScaling=2^0
  RMS : Outport  Port=4  OutDataType=fixdt(1, 16)  OutScaling=2^0
  freq : Outport  Port=5  OutDataType=fixdt(1, 16)  OutScaling=2^0
  Pmm : Outport  Port=6
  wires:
  E_req/1 -> UWM_controller/3(E_req)
  P_req/1 -> UWM_controller/4(P_req)
  Three-Phase V-I Measurement/1 -> UWM_controller/1(v_meas), 3-phase  Instantaneous  Active & Reactive Power/1, RMS block1/1, V/1
  Three-Phase V-I Measurement/2 -> UWM_controller/2(i_meas), 3-phase  Instantaneous  Active & Reactive Power/2, RMS block/1, I/1
  UWM_controller/1(Vpk) -> microsource/1(Vpk)
  UWM_controller/2(w) -> microsource/2(w), Gain/1
  Gain/1 -> freq/1
  3-phase  Instantaneous  Active & Reactive Power/1 -> PQ/1
  RMS block1/1 -> Mux/1
  RMS block/1 -> Mux/2
  Mux/1 -> RMS/1
  UWM_controller/3(Pmm) -> Pmm/1
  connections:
  b/RConn1 -- Three-Phase V-I Measurement/RConn2
  Three-Phase V-I Measurement/RConn3 -- c/RConn1
  10 mH/LConn2 -- microsource/RConn2
  10 mH/LConn1 -- microsource/RConn1
  10 mH/LConn3 -- microsource/RConn3
  T1/LConn1 -- 10 mH/RConn1
  T1/LConn2 -- 10 mH/RConn2
  T1/LConn3 -- 10 mH/RConn3
  T1/RConn1 -- Three-Phase V-I Measurement/LConn1
  T1/RConn2 -- Three-Phase V-I Measurement/LConn2
  T1/RConn3 -- Three-Phase V-I Measurement/LConn3
  a/RConn1 -- Three-Phase V-I Measurement/RConn1

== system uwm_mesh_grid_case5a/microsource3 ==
  E_req : Inport
  P_req : Inport  Port=2
  10 mH : powerlib/Elements/Three-Phase Series RLC Branch  DialogController=POWERSYS.PowerSysDialog  PhysicalDomain=powersysdomain  SubClassName=unknown  LeftPortType=p1  RightPortType=p1  LConnTagsString=A|B|C  RConnTagsString=A|B|C  BranchType=L  Resistance=.0028  Inductance=5e-3  Capacitance=1e-6  Measurements=None
  3-phase  Instantaneous  Active & Reactive Power : powerlib_extras/Measurements/3-phase  Instantaneous  Active & Reactive Power  DialogController=POWERSYS.PowerSysDialog  SystemSampleTime=-1
  Gain : Gain  Gain=1/(2*pi)  ParameterDataType=fixdt(1, 16)  ParameterScaling=2^0  OutDataType=fixdt(1, 16)  OutScaling=2^0
  Mux : Mux  Inputs=2
  RMS block : Fcn  Expr=sqrt(u(1)*u(1)+u(2)*u(2)+u(3)*u(3))/sqrt(3)
  RMS block1 : Fcn  Expr=sqrt(u(1)*u(1)+u(2)*u(2)+u(3)*u(3))/sqrt(3)
  T1 : powerlib/Elements/Three-Phase Transformer (Two Windings)  DialogController=POWERSYS.PowerSysDialog  SystemSampleTime=-1  Winding1Connection=Delta (D1)  UNITS=SI  NominalPower=[ 45e3 , 60 ]  Winding1=[208 0.02688 0.1075/(2*pi*60)]  Winding2Connection=Yg  Winding2=[208 0.005047 .0201/(2*pi*60)]  SetSaturation=off  Rm=100.e6  Lm=7650.8  Saturation=[0 0;1359.8 0.93633;5.6659e+05 1.186]  Hysteresis=off  DataFile='hysteresis'  SetInitialFlux=off  InitialFluxes=[0.62422 -0.62422 0.54618]  Measurements=None  MoreParameters=off  BreakLoop=off  DataType=on  TransfoNumber=1
  Three-Phase V-I Measurement : powerlib/Measurements/Three-Phase V-I Measurement  DialogController=POWERSYS.PowerSysDialog  SystemSampleTime=-1  VoltageMeasurement=phase-to-ground  SetLabelV=off  LabelV=Vabc  Vpu=off  VpuLL=off  CurrentMeasurement=yes  SetLabelI=off  LabelI=Iabc  Ipu=off  Pbase=100e6  Vbase=500e3  OutputType=Complex  PhasorSimulation=off  PSBequivalent=0
  UWM_controller : Subsystem  mask{Vbase=208, Sbase=15000}
  microsource : Subsystem
  a : PMIOPort  Port=1  Side=Right
  b : PMIOPort  Port=2  Side=Right
  c : PMIOPort  Port=3  Side=Right
  PQ : Outport  OutDataType=fixdt(1, 16)  OutScaling=2^0
  V : Outport  Port=2  OutDataType=fixdt(1, 16)  OutScaling=2^0
  I : Outport  Port=3  OutDataType=fixdt(1, 16)  OutScaling=2^0
  RMS : Outport  Port=4  OutDataType=fixdt(1, 16)  OutScaling=2^0
  freq : Outport  Port=5  OutDataType=fixdt(1, 16)  OutScaling=2^0
  Pmm : Outport  Port=6
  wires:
  E_req/1 -> UWM_controller/3(E_req)
  P_req/1 -> UWM_controller/4(P_req)
  Three-Phase V-I Measurement/1 -> UWM_controller/1(v_meas), 3-phase  Instantaneous  Active & Reactive Power/1, RMS block1/1, V/1
  Three-Phase V-I Measurement/2 -> UWM_controller/2(i_meas), 3-phase  Instantaneous  Active & Reactive Power/2, RMS block/1, I/1
  UWM_controller/1(Vpk) -> microsource/1(Vpk)
  UWM_controller/2(w) -> microsource/2(w), Gain/1
  Gain/1 -> freq/1
  3-phase  Instantaneous  Active & Reactive Power/1 -> PQ/1
  RMS block1/1 -> Mux/1
  RMS block/1 -> Mux/2
  Mux/1 -> RMS/1
  UWM_controller/3(Pmm) -> Pmm/1
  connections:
  b/RConn1 -- Three-Phase V-I Measurement/RConn2
  Three-Phase V-I Measurement/RConn3 -- c/RConn1
  10 mH/LConn2 -- microsource/RConn2
  10 mH/LConn1 -- microsource/RConn1
  10 mH/LConn3 -- microsource/RConn3
  T1/LConn1 -- 10 mH/RConn1
  T1/LConn2 -- 10 mH/RConn2
  T1/LConn3 -- 10 mH/RConn3
  T1/RConn1 -- Three-Phase V-I Measurement/LConn1
  T1/RConn2 -- Three-Phase V-I Measurement/LConn2
  T1/RConn3 -- Three-Phase V-I Measurement/LConn3
  a/RConn1 -- Three-Phase V-I Measurement/RConn1

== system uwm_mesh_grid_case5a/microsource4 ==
  E_req : Inport
  P_req : Inport  Port=2
  10 mH : powerlib/Elements/Three-Phase Series RLC Branch  DialogController=POWERSYS.PowerSysDialog  PhysicalDomain=powersysdomain  SubClassName=unknown  LeftPortType=p1  RightPortType=p1  LConnTagsString=A|B|C  RConnTagsString=A|B|C  BranchType=L  Resistance=.0028  Inductance=5e-3  Capacitance=1e-6  Measurements=None
  3-phase  Instantaneous  Active & Reactive Power : powerlib_extras/Measurements/3-phase  Instantaneous  Active & Reactive Power  DialogController=POWERSYS.PowerSysDialog  SystemSampleTime=-1
  Gain : Gain  Gain=1/(2*pi)  ParameterDataType=fixdt(1, 16)  ParameterScaling=2^0  OutDataType=fixdt(1, 16)  OutScaling=2^0
  Mux : Mux  Inputs=2
  RMS block : Fcn  Expr=sqrt(u(1)*u(1)+u(2)*u(2)+u(3)*u(3))/sqrt(3)
  RMS block1 : Fcn  Expr=sqrt(u(1)*u(1)+u(2)*u(2)+u(3)*u(3))/sqrt(3)
  T1 : powerlib/Elements/Three-Phase Transformer (Two Windings)  DialogController=POWERSYS.PowerSysDialog  SystemSampleTime=-1  Winding1Connection=Delta (D1)  UNITS=SI  NominalPower=[ 45e3 , 60 ]  Winding1=[208 0.02688 0.1075/(2*pi*60)]  Winding2Connection=Yg  Winding2=[208 0.005047 .0201/(2*pi*60)]  SetSaturation=off  Rm=100.e6  Lm=7650.8  Saturation=[0 0;1359.8 0.93633;5.6659e+05 1.186]  Hysteresis=off  DataFile='hysteresis'  SetInitialFlux=off  InitialFluxes=[0.62422 -0.62422 0.54618]  Measurements=None  MoreParameters=off  BreakLoop=off  DataType=on  TransfoNumber=1
  Three-Phase V-I Measurement : powerlib/Measurements/Three-Phase V-I Measurement  DialogController=POWERSYS.PowerSysDialog  SystemSampleTime=-1  VoltageMeasurement=phase-to-ground  SetLabelV=off  LabelV=Vabc  Vpu=off  VpuLL=off  CurrentMeasurement=yes  SetLabelI=off  LabelI=Iabc  Ipu=off  Pbase=100e6  Vbase=500e3  OutputType=Complex  PhasorSimulation=off  PSBequivalent=0
  UWM_controller : Subsystem  mask{Vbase=208, Sbase=15000}
  microsource : Subsystem
  a : PMIOPort  Port=1  Side=Right
  b : PMIOPort  Port=2  Side=Right
  c : PMIOPort  Port=3  Side=Right
  PQ : Outport  OutDataType=fixdt(1, 16)  OutScaling=2^0
  V : Outport  Port=2  OutDataType=fixdt(1, 16)  OutScaling=2^0
  I : Outport  Port=3  OutDataType=fixdt(1, 16)  OutScaling=2^0
  RMS : Outport  Port=4  OutDataType=fixdt(1, 16)  OutScaling=2^0
  freq : Outport  Port=5  OutDataType=fixdt(1, 16)  OutScaling=2^0
  Pmm : Outport  Port=6
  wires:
  E_req/1 -> UWM_controller/3(E_req)
  P_req/1 -> UWM_controller/4(P_req)
  Three-Phase V-I Measurement/1 -> UWM_controller/1(v_meas), 3-phase  Instantaneous  Active & Reactive Power/1, RMS block1/1, V/1
  Three-Phase V-I Measurement/2 -> UWM_controller/2(i_meas), 3-phase  Instantaneous  Active & Reactive Power/2, RMS block/1, I/1
  UWM_controller/1(Vpk) -> microsource/1(Vpk)
  UWM_controller/2(w) -> microsource/2(w), Gain/1
  Gain/1 -> freq/1
  3-phase  Instantaneous  Active & Reactive Power/1 -> PQ/1
  RMS block1/1 -> Mux/1
  RMS block/1 -> Mux/2
  Mux/1 -> RMS/1
  UWM_controller/3(Pmm) -> Pmm/1
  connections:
  b/RConn1 -- Three-Phase V-I Measurement/RConn2
  Three-Phase V-I Measurement/RConn3 -- c/RConn1
  10 mH/LConn2 -- microsource/RConn2
  10 mH/LConn1 -- microsource/RConn1
  10 mH/LConn3 -- microsource/RConn3
  T1/LConn1 -- 10 mH/RConn1
  T1/LConn2 -- 10 mH/RConn2
  T1/LConn3 -- 10 mH/RConn3
  T1/RConn1 -- Three-Phase V-I Measurement/LConn1
  T1/RConn2 -- Three-Phase V-I Measurement/LConn2
  T1/RConn3 -- Three-Phase V-I Measurement/LConn3
  a/RConn1 -- Three-Phase V-I Measurement/RConn1
